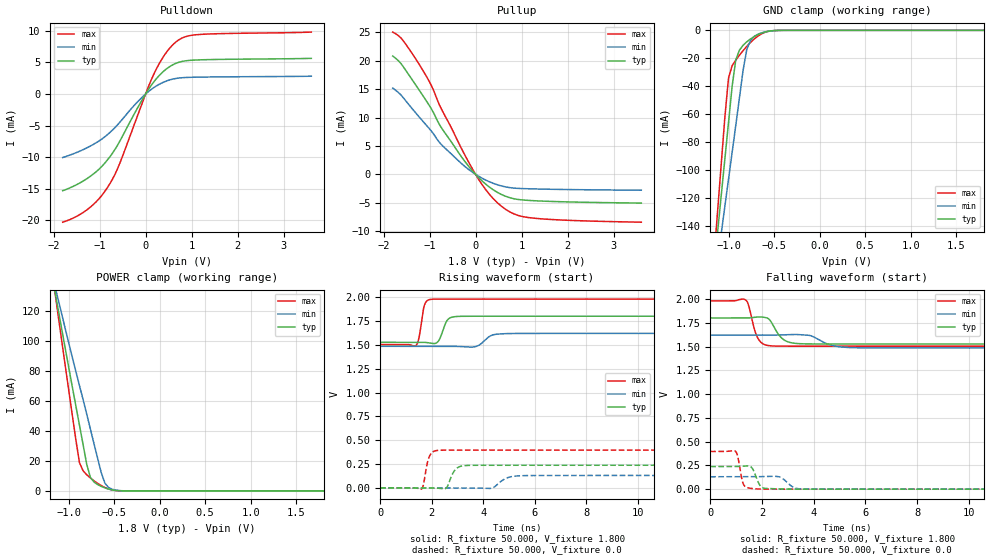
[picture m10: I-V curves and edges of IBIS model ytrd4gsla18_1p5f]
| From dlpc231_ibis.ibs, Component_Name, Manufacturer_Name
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| Model ytrd4gsla18_1p5f
[Model] ytrd4gsla18_1p5f
Model_type 3-state
Polarity   Non-Inverting
Enable   Active-High
Vmeas =  0.900V
Cref =  50.000pF
Rref =  0.500k
Vref =  0.0V
C_comp   1.638pF   1.512pF   1.774pF
C_comp_pullup   0.870pF   0.789pF   0.960pF
C_comp_pulldown   0.870pF   0.789pF   0.960pF
[Temperature Range]   25.000   0.125k   -40.000
[Voltage Range]   1.800V   1.620V   1.980V
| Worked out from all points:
|   slope of the pulldown table from 0 to 0.27 V, typ, clamps not added: 99.4 ohm
|   slope of the pullup table from 0 to 0.27 V, typ, clamps not added: 132 ohm
|   GND clamp passes 1 mA (typ) near -0.59 V on its own axis
|   POWER clamp passes 1 mA (typ) near -0.54 V on its own axis
|   rising waveform, R_fixture 50.000, V_fixture 1.800: 20-80 % time 231ps typ, 356ps min, 163ps max; typ from 1.53 V to 1.8 V
|   rising waveform, R_fixture 50.000, V_fixture 0.0: 20-80 % time 252ps typ, 413ps min, 180ps max; typ from 0 V to 0.238 V
|   falling waveform, R_fixture 50.000, V_fixture 1.800: 20-80 % time 410ps typ, 651ps min, 289ps max; typ from 1.8 V to 1.53 V
|   falling waveform, R_fixture 50.000, V_fixture 0.0: 20-80 % time 219ps typ, 335ps min, 163ps max; typ from 0.238 V to 0 V
[Pulldown]
-1.8V     -15.3mA    -10.05mA   -20.28mA
-1.2V     -13.02mA   -8.229mA   -17.9mA
-960mV    -11.53mA   -7.177mA   -16.13mA
-780mV    -9.975mA   -6.114mA   -14.25mA
-540mV    -7.195mA   -4.305mA   -10.6mA
-120mV    -1.499mA   -829uA     -2.359mA
180mV     1.936mA    1.026mA    3.159mA
420mV     3.782mA    1.968mA    6.273mA
660mV     4.863mA    2.466mA    8.245mA
840mV     5.225mA    2.604mA    9.012mA
1.14V     5.399mA    2.671mA    9.408mA
3.6V      5.646mA    2.818mA    9.802mA
[Pullup]
-1.8V     20.84mA    15.19mA    25.06mA
-1.56V    18.83mA    13.39mA    23.42mA
-1.08V    13.06mA    8.751mA    17.43mA
-960mV    11.53mA    7.619mA    15.65mA
-720mV    7.931mA    5.047mA    11.15mA
-180mV    1.72mA     1.042mA    2.588mA
60mV      -515.7uA   -302.6uA   -801.4uA
240mV     -1.861mA   -1.088mA   -2.907mA
600mV     -3.691mA   -2.122mA   -5.865mA
900mV     -4.402mA   -2.466mA   -7.176mA
1.26V     -4.645mA   -2.568mA   -7.72mA
3.6V      -5.067mA   -2.799mA   -8.432mA
[GND_clamp]
-1.8V     -597.4mA   -500.9mA   -710mA
-1.16V    -170.9mA   -184.3mA   -163.5mA
-1.12V    -144.6mA   -164.8mA   -129.7mA
-1.08V    -118.4mA   -145.4mA   -95.95mA
-1.04V    -92.22mA   -126mA     -62.27mA
-1V       -66.09mA   -106.6mA   -34.11mA
-960mV    -39.93mA   -87.3mA    -25.33mA
-920mV    -21.05mA   -67.84mA   -21.23mA
-800mV    -8.254mA   -13.78mA   -11.5mA
-680mV    -3.146mA   -2.862mA   -4.259mA
-440mV    -43.6uA    -64.31uA   -34.79uA
1.8V      0A         0A         0A
[POWER_clamp]
-1.8V     367.9mA    313.2mA    432.7mA
-1.16V    136.5mA    139.2mA    137mA
-1.12V    123mA      129mA      119.6mA
-920mV    56.74mA    79.65mA    34.28mA
-880mV    43.81mA    70.18mA    18.86mA
-840mV    30.81mA    60.69mA    13.38mA
-800mV    17.64mA    50.99mA    10.77mA
-760mV    9.019mA    41.18mA    8.633mA
-680mV    4.212mA    21.63mA    4.996mA
-600mV    1.988mA    5.044mA    2.281mA
-480mV    292.3uA    521.1uA    246.1uA
1.8V      0A         0A         0A
[Ramp]
dV/dt_r 0.143/0.251n   78.317m/0.415n   0.238/0.183n
dV/dt_f 0.164/0.417n   81.123m/0.657n   0.286/0.295n
R_load = 50.000
[Rising Waveform]
R_fixture= 50.000
V_fixture= 1.800
V_fixture_min= 1.620
V_fixture_max= 1.980
0s        1.527V     1.485V     1.503V
1.388ns   1.527V     1.485V     1.493V
1.508ns   1.527V     1.485V     1.58V
1.718ns   1.526V     1.485V     1.919V
1.958ns   1.518V     1.485V     1.977V
2.239ns   1.533V     1.485V     1.98V
2.599ns   1.757V     1.485V     1.98V
2.947ns   1.797V     1.484V     1.98V
4.812ns   1.8V       1.617V     1.98V
15ns      1.8V       1.62V      1.98V
[Rising Waveform]
R_fixture= 50.000
V_fixture= 0.0
V_fixture_min= 0.0
V_fixture_max= 0.0
0s        0V         0V         0V
1.608ns   15.97uV    0V         -11.47mV
1.908ns   413.1uV    -931.8nV   330.5mV
2.238ns   -2.531mV   -2.969uV   393.6mV
2.559ns   -2.439mV   -1.318uV   396.2mV
2.899ns   186.9mV    83.63uV    396.4mV
3.311ns   234.7mV    270.7uV    396.4mV
4.322ns   237.6mV    -3.356mV   396.4mV
5.402ns   237.6mV    127.2mV    396.4mV
15ns      237.6mV    130.5mV    396.4mV
[Falling Waveform]
R_fixture= 50.000
V_fixture= 1.800
V_fixture_min= 1.620
V_fixture_max= 1.980
0s        1.8V       1.62V      1.98V
1.379ns   1.8V       1.62V      1.987V
1.478ns   1.8V       1.62V      1.937V
1.699ns   1.807V     1.62V      1.689V
1.83ns    1.81V      1.62V      1.593V
2.289ns   1.783V     1.62V      1.508V
2.779ns   1.585V     1.623V     1.504V
3.359ns   1.531V     1.626V     1.503V
5.379ns   1.527V     1.489V     1.503V
15ns      1.527V     1.485V     1.503V
[Falling Waveform]
R_fixture= 50.000
V_fixture= 0.0
V_fixture_min= 0.0
V_fixture_max= 0.0
0s        237.6mV    130.5mV    396.4mV
979ps     238.2mV    130.5mV    396.8mV
1.069ns   238.8mV    130.5mV    335.3mV
1.279ns   242mV      130.5mV    54.31mV
1.679ns   192.6mV    130.9mV    4.951mV
1.929ns   36.4mV     131.6mV    1.146mV
2.169ns   7.45mV     133.1mV    251.4uV
2.697ns   2.305mV    126.9mV    8.692uV
3.489ns   85.67uV    3.536mV    0V
15ns      0V         0V         0V
